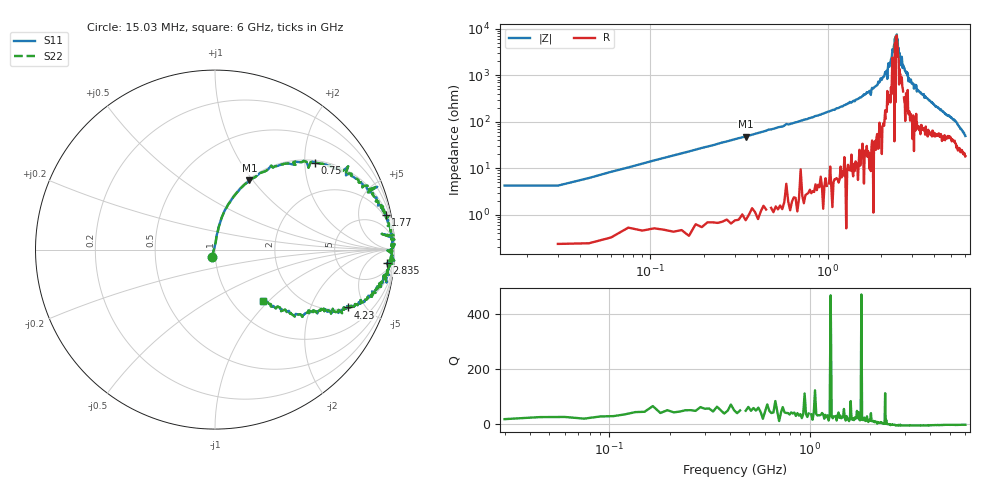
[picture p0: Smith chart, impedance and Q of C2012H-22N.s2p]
!	Network	Analyzer	HP8753E.07.74:	Oct	30	2002	Serial	No.	JP38451487
!	Hewlett-Packard
!	28	Aug	2009	9:53:35
!	Frequency	S11	S21	S12	S22
#	HZ	S	RI	R	50
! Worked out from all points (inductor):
!   400 points, 15.03 MHz to 6 GHz, reference 50 ohm
!   read as one part in series: L = 22.1 nH near 45.03 MHz
!   highest Q = 55.5 at 345 MHz (marker M1), where L = 22.2 nH
!   self-resonance near 2.43 GHz
!   S11 on the Smith chart (normalised r, x): 15.03 MHz: 0.96, -0.08; 750 MHz: 1.05, +2.25; 1.77 GHz: 1.57, +9.80; 2.835 GHz: 11, -20; 4.23 GHz: 2.03, -3.77; 6 GHz: 1.36, -0.92
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1.502992e7  -0.0163 -0.0394  1.02 0.0394  1.02 0.0394  -0.0163 -0.0394
1.350293e8  0.038 0.18  0.962 -0.18  0.962 -0.18  0.038 0.18
3.450283e8  0.192 0.386  0.808 -0.386  0.808 -0.386  0.192 0.386
7.500262e8  0.558 0.485  0.442 -0.485  0.442 -0.485  0.558 0.485
1.020025e9  0.73 0.43  0.27 -0.43  0.27 -0.43  0.73 0.43
1.770021e9  0.95 0.191  0.0501 -0.191  0.0501 -0.191  0.95 0.191
2.01002e9  0.977 0.122  0.0235 -0.122  0.0235 -0.122  0.977 0.122
2.175019e9  0.929 0.0875  0.0705 -0.0875  0.0705 -0.0875  0.929 0.0875
2.400018e9  0.987 0.00983  0.0127 -0.00983  0.0127 -0.00983  0.987 0.00983
2.415018e9  0.998 0.0253  0.00232 -0.0253  0.00232 -0.0253  0.998 0.0253
2.430018e9  0.986 0.00394  0.0136 -0.00394  0.0136 -0.00394  0.986 0.00394
2.445018e9  0.973 -0.00583  0.0269 0.00583  0.0269 0.00583  0.973 -0.00583
2.460018e9  0.987 -0.00409  0.0125 0.00409  0.0125 0.00409  0.987 -0.00409
2.490018e9  0.988 -0.0119  0.0119 0.0119  0.0119 0.0119  0.988 -0.0119
2.505017e9  0.961 -0.00497  0.0386 0.00497  0.0386 0.00497  0.961 -0.00497
2.520017e9  0.984 -0.0202  0.0156 0.0202  0.0156 0.0202  0.984 -0.0202
2.835016e9  0.957 -0.0746  0.0432 0.0746  0.0432 0.0746  0.957 -0.0746
3.015015e9  0.97 -0.141  0.0296 0.141  0.0296 0.141  0.97 -0.141
4.00501e9  0.794 -0.31  0.206 0.31  0.206 0.31  0.794 -0.31
4.230009e9  0.741 -0.322  0.259 0.322  0.259 0.322  0.741 -0.322
5.010005e9  0.575 -0.343  0.425 0.343  0.425 0.343  0.575 -0.343
6e9  0.265 -0.286  0.735 0.286  0.735 0.286  0.265 -0.286
